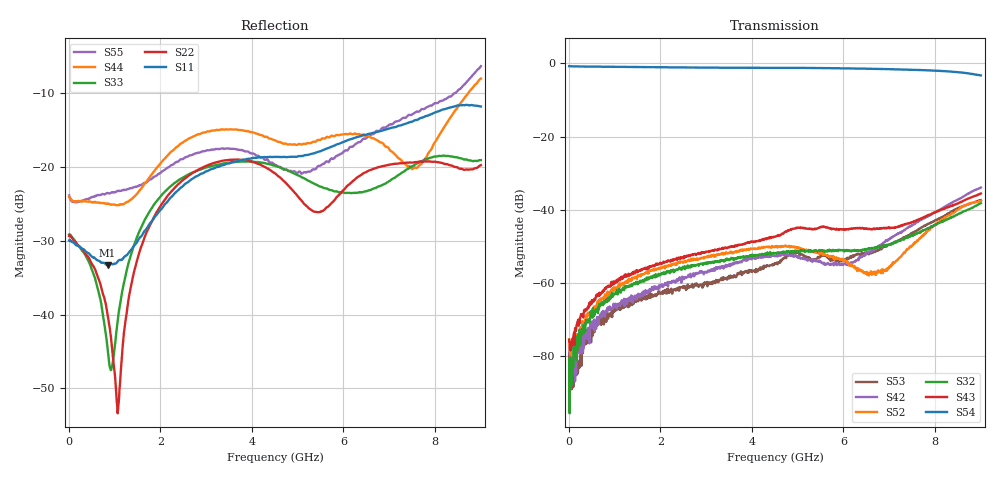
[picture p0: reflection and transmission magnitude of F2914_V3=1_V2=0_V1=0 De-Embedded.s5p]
! Integrated Device Technology
! Corporate Headquarters
! 6024 Silver Creek Valley Road
! San Jose, CA 95138  USA
! Phone:  1-408-284-8200
! Toll Free:  1-800-223-1366
! Webpage:  http://www.idt.com/
! Timing and RF Division
! 515 Groton Road, Suite 102
! Westford, MA 01886-6024
! Device:  F2914
! Description: High Reliability SP4T RF Switch
! Frequency:  0.05 -  8.GHz
! Package:  4x4 mm Thin QFN Plastic Package: 24 pin
! Ports:  5 RF,  5 DC
!  Pin  1  = GND
!  Pin  2  = GND
!  Pin  3  = GND
!  Pin  4  = GND
!  Pin  5  = RF4  =  Port 4
!  Pin  6  = GND
!  Pin  7  = GND
!  Pin  8  = RF3  =  Port 3
!  Pin  9  = GND
!  Pin 10  = GND
!  Pin 11  = RF2  =  Port 2
!  Pin 12  = GND
!  Pin 13  = GND
!  Pin 14  = RF1  =  Port 1
!  Pin 15  = GND
!  Pin 16  = Vcc
!  Pin 17  = V1
!  Pin 18  = V2
!  Pin 19  = V3
!  Pin 20  = VSSext
!  Pin 21  = GND
!  Pin 22  = RFC  =  Port 5
!  Pin 23  = GND
!  Pin 24  = GND
! Voltage:  VDD  =  +3.30 Volts
!  VSSEXT =  0.00 Volts
! Current:  IDD  = 325  uA
! State:  RF4 Selected
! V1:  Logic LOW
! V2:  Logic LOW
! V3:  Logic HIGH
! Data:  The device was measured on the F291x evaluation board which has
!  individual transmission lines to the RF pins.  Data was collected
!  using a calibrated network analyzer.  The input lines were
!  modeled using Automatic Fixture Removal (AFR) from Keysight.
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# Hz S  dB  R 50
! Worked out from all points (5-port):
!   900 points, 10 MHz to 9 GHz, reference 50 ohm
!   strongest paths, dB at 10 MHz, 2.26 GHz, 4.51 GHz, 6.76 GHz, 9 GHz:
!     S54: -0.8, -1.1, -1.2, -1.5, -3.3
!     S43: -75.4, -53.6, -47.3, -45.2, -35.5
!     S32: -80.8, -56.6, -51.8, -50.1, -38.2
!     S52: -75.3, -55.0, -50.0, -56.5, -37.5
!     S42: -76.8, -59.4, -52.7, -50.2, -33.9
!     S53: -80.1, -62.9, -54.7, -51.1, -37.4
!   lowest |S11| = -33.3 dB at 850 MHz (marker M1), VSWR 1.04, Z = 48.6 + j1.6 ohm
!   |S11| at or under -10 dB: start of sweep to end of sweep
